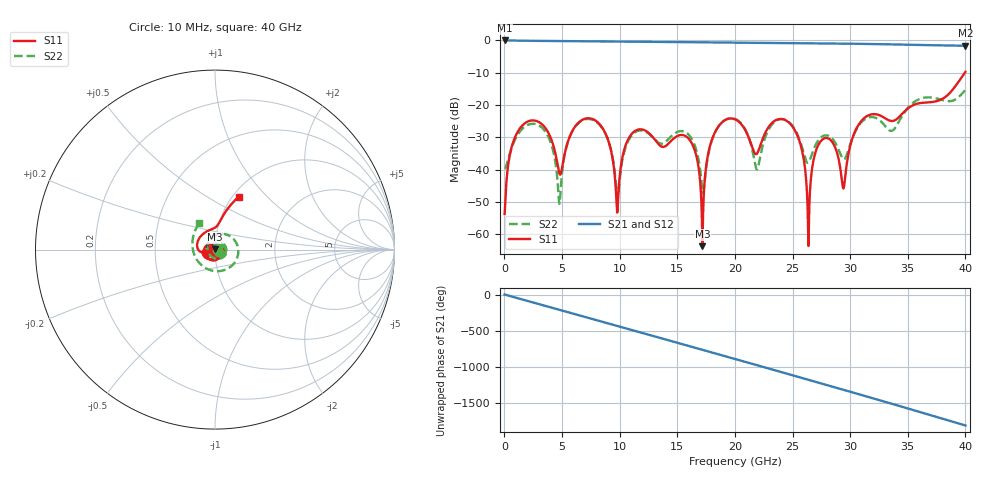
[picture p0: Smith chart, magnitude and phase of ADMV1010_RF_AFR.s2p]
! Analog Devices, Inc.
! 1 Analog Way
! Wilmington, MA 01887
! http://www.analog.com
! Date:  2021-09-07 NN
! Board Name:  ADMV1010-EVALZ Revision B with ADMV1010AEZ installed
! File Description:  Automatic Fixture Removal S-Parameters for RF Port connector and board loss de-embedding
! File Generation:  Calibrated Network Analyzer
! Chip Part Number:  ADMV1010
! Chip Description:  GaAs, MMIC, IQ Downconverter
! Chip Frequency:  12.6 to 15.4 GHz
! Chip Package:  LCC, 4.9 x 4.9 x 1 mm
! RF Port:  ADMV1010AEZ removed and end of trace left open
! Note:
!  Analog Devices supplies this data as a sample of measured data at the evaluation board
!  ports for this product.  Your particular data for this product may vary.
!  Analog Devices reserves the right to change this data at anytime.
!  All lines below in this file are as is from the Network Analyzer.
!Agilent Technologies,N5245A,MY52451809,A.10.47.06
!Automatic Fixture Removal (AFR)
!Date: Friday, August 27, 2021 5:30:25 AM
!S2P File: Measurements: S11,S21,S12,S22:
# MHz S  RI  R 50
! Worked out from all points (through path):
!   4000 points, 10 MHz to 40 GHz, reference 50 ohm
!   highest |S21| = 0.00 dB at 10 MHz (marker M1); lowest = -1.6 dB at 40 GHz (marker M2)
!   group delay of S21, straight-line fit = 126 ps
!   lowest |S11| = -63.7 dB at 17.18 GHz (marker M3), VSWR 1.00, Z = 50 + j0.061 ohm
!   |S11| at or under -10 dB: start of sweep to 39.95 GHz
!   |S22| runs from -50.6 to -15.3 dB; largest |S21 - S12| = 1.4e-15
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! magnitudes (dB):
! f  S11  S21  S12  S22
! 10 MHz  -53.7  0.0  0.0  -39.7
! 1.52 GHz  -26.4  -0.1  -0.1  -27.5
! 3.63 GHz  -27.5  -0.2  -0.2  -28.7
! 4.77 GHz  -41.3  -0.2  -0.2  -50.6
! 6.68 GHz  -24.7  -0.3  -0.3  -24.9
! 8.73 GHz  -28.6  -0.3  -0.3  -28.7
! 9.78 GHz  -53.3  -0.3  -0.3  -48.5
! 11.01 GHz  -29.1  -0.4  -0.4  -29.6
! 13.34 GHz  -32.0  -0.5  -0.5  -31.6
! 16.08 GHz  -30.8  -0.5  -0.5  -29.6
! 17.18 GHz  -63.7  -0.6  -0.6  -46.3
! 18.09 GHz  -29.9  -0.6  -0.6  -30.0
! 20.01 GHz  -24.4  -0.7  -0.7  -24.3
! 21.89 GHz  -35.1  -0.7  -0.7  -39.9
! 24.28 GHz  -24.5  -0.8  -0.8  -24.5
! 25.67 GHz  -32.0  -0.9  -0.9  -31.4
! 26.35 GHz  -59.2  -0.9  -0.9  -37.9
! 26.67 GHz  -40.3  -0.9  -0.9  -35.3
! 28.03 GHz  -30.3  -0.9  -0.9  -29.4
! 29.42 GHz  -45.8  -1.0  -1.0  -36.8
! 33.34 GHz  -24.7  -1.2  -1.2  -27.7
! 40 GHz  -9.7  -1.6  -1.6  -15.3
